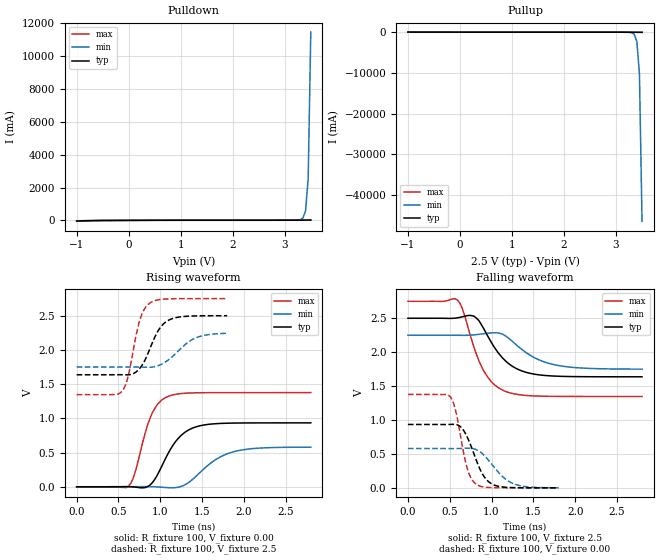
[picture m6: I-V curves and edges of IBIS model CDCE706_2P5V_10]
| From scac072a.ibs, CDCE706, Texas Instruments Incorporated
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|   Model   CDCE706_2P5V_10
[Model]   CDCE706_2P5V_10
Model_type   Output
Polarity   Non-Inverting
Vmeas  =   1.50V
Cref   =   3.00pF
Rref   =   100
Vref   =   0.00V
|Variable   typ   min   max
C_comp   1.510e-12   1.502e-12   1.531e-12
|Variable   typ   min   max
[Voltage range]   2.5   2.25   2.75
|Variable   typ   min   max
[Temperature range]  55   110   -15
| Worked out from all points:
|   slope of the pulldown table from 0 to 0.375 V, typ, clamps not added: 94 ohm
|   slope of the pullup table from 0 to 0.375 V, typ, clamps not added: 111 ohm
|   rising waveform, R_fixture 100, V_fixture 0.00: 20-80 % time 275ps typ, 371ps min, 200ps max; typ from 0 V to 0.934 V
|   falling waveform, R_fixture 100, V_fixture 2.5: 20-80 % time 314ps typ, 389ps min, 262ps max; typ from 2.5 V to 1.64 V
|   rising waveform, R_fixture 100, V_fixture 2.5: 20-80 % time 202ps typ, 283ps min, 146ps max; typ from 1.64 V to 2.5 V
|   falling waveform, R_fixture 100, V_fixture 0.00: 20-80 % time 191ps typ, 258ps min, 135ps max; typ from 0.935 V to 0 V
[Pulldown]
|Voltage   I(typ)   I(min)   I(max)
-1V       -42.02mA   -49.47mA   -54.59mA
200mV     2.308mA    1.463mA    3.645mA
3.15V     11.36mA    11.49mA    14.95mA
3.3V      14.88mA    48.65mA    16.39mA
3.35V     16.25mA    150mA      17.66mA
3.4V      17.76mA    588.5mA    19.13mA
3.45V     19.65mA    2.556A     20.75mA
3.5V      23.13mA    11.48A     22.52mA
[Pullup]
|Voltage   I(typ)   I(min)   I(max)
-1V       22.36mA    22.42mA    30.24mA
3.15V     -14.4mA    -19.41mA   -16.98mA
3.3V      -22.2mA    -139.3mA   -19.18mA
3.35V     -25.42mA   -531.5mA   -21.34mA
3.4V      -28.99mA   -2.29A     -24.19mA
3.45V     -33.43mA   -10.26A    -27.6mA
3.5V      -41.93mA   -46.45A    -31.47mA
[Ramp]
|Variable   typ   min   max
dV/dt_r  0.2947/2.210e-10   0.1770/3.152e-10   0.4770/1.632e-10
dV/dt_f  0.2638/2.444e-10   0.1519/3.285e-10   0.4362/1.902e-10
R_load  =  50
[Rising Waveform]
R_fixture   =   100
V_fixture   =   0.00
V_fixture_min   =   0.00
V_fixture_max   =   0.00
C_fixture   =   0.00
|Time   V(typ)   V(min)   V(max)
0s        0V         0V         0V
622.2ps   2.045mV    46.62uV    11.23mV
678.8ps   -1.829mV   426uV      135.6mV
848.5ps   1.64mV     2.076mV    906.9mV
905.1ps   59.4mV     771.2uV    1.082V
1.075ns   442.5mV    -11.81mV   1.311V
1.244ns   744.9mV    3.316mV    1.362V
1.471ns   890.1mV    203.6mV    1.374V
1.895ns   931mV      517.2mV    1.375V
2.8ns     933.8mV    578.8mV    1.376V
[Falling Waveform]
R_fixture   =   100
V_fixture   =   2.5
V_fixture_min   =   2.25
V_fixture_max   =   2.75
C_fixture   =   0.00
|Time   V(typ)   V(min)   V(max)
0s        2.5V       2.25V      2.75V
593.9ps   2.507V     2.249V     2.766V
650.5ps   2.521V     2.248V     2.643V
791.9ps   2.529V     2.255V     2.064V
905.1ps   2.351V     2.272V     1.729V
1.018ns   2.102V     2.286V     1.539V
1.16ns    1.881V     2.245V     1.426V
1.386ns   1.714V     2.019V     1.365V
1.725ns   1.649V     1.823V     1.349V
2.8ns     1.637V     1.75V      1.347V
[Rising Waveform]
R_fixture   =   100
V_fixture   =   2.5
V_fixture_min   =   2.25
V_fixture_max   =   2.75
C_fixture   =   0.00
|Time   V(typ)   V(min)   V(max)
0s        1.636V     1.749V     1.346V
545.5ps   1.637V     1.749V     1.402V
618.2ps   1.636V     1.749V     1.627V
709.1ps   1.676V     1.75V      2.203V
763.6ps   1.745V     1.749V     2.466V
890.9ps   2.063V     1.747V     2.696V
1ns       2.327V     1.782V     2.736V
1.127ns   2.449V     1.883V     2.746V
1.418ns   2.496V     2.172V     2.749V
1.8ns     2.499V     2.243V     2.749V
[Falling Waveform]
R_fixture   =   100
V_fixture   =   0.00
V_fixture_min   =   0.00
V_fixture_max   =   0.00
C_fixture   =   0.00
|Time   V(typ)   V(min)   V(max)
0s        934.5mV    579.9mV    1.377V
509.1ps   935.5mV    579mV      1.342V
581.8ps   931.7mV    579.2mV    1.084V
672.7ps   834.1mV    583mV      476.5mV
727.3ps   699.2mV    584.4mV    217.5mV
836.4ps   348.4mV    552.6mV    38.7mV
909.1ps   169.6mV    482.8mV    12.76mV
981.8ps   74.94mV    380.5mV    4.83mV
1.236ns   4.656mV    75.51mV    799.9uV
1.8ns     489.1uV    1.355mV    526.7uV
